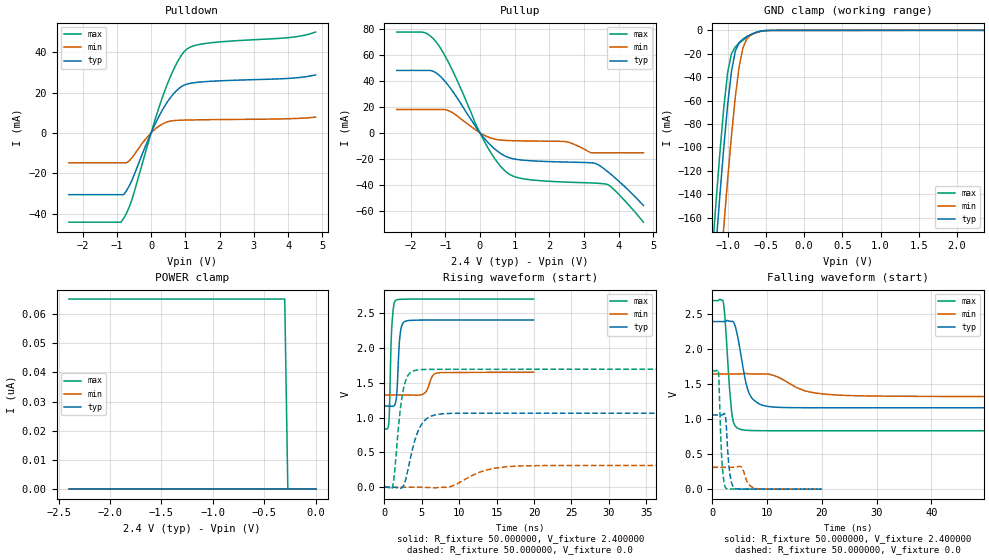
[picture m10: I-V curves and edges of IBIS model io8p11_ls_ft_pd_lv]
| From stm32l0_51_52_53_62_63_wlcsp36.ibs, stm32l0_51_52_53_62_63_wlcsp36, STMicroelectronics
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|   Model io8p11_ls_ft_pd_lv
[Model]  io8p11_ls_ft_pd_lv
Model_type I/O
Polarity   Non-Inverting
Enable   Active-Low
Vinl =   0.720000V
Vinh =   1.680000V
Vmeas =  1.200000V
Cref =   50.000000pF
Rref =   100.000000M
Vref =   0.0V
C_comp   4.521100pF   4.438000pF   4.578000pF
[Temperature Range]   25.000000   0.105000k   -40.000000
[Pullup Reference]   2.400000V   1.650000V   2.700000V
[Pulldown Reference]   0.0V   0.0V   0.0V
[POWER Clamp Reference]   2.400000V   1.650000V   2.700000V
[GND Clamp Reference]   0.0V   0.0V   0.0V
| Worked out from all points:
|   slope of the pulldown table from 0 to 0.36 V, typ, clamps not added: 29.5 ohm
|   slope of the pullup table from 0 to 0.36 V, typ, clamps not added: 33.2 ohm
|   GND clamp passes 1 mA (typ) near -0.59 V on its own axis
|   rising waveform, R_fixture 50.000000, V_fixture 2.400000: 20-80 % time 365ps typ, 690ps min, 304ps max; typ from 1.17 V to 2.4 V
|   rising waveform, R_fixture 50.000000, V_fixture 0.0: 20-80 % time 1.62ns typ, 3.85ns min, 984ps max; typ from 0 V to 1.06 V
|   falling waveform, R_fixture 50.000000, V_fixture 2.400000: 20-80 % time 1.82ns typ, 5.41ns min, 983ps max; typ from 2.4 V to 1.17 V
|   falling waveform, R_fixture 50.000000, V_fixture 0.0: 20-80 % time 621ps typ, 1.01ns min, 515ps max; typ from 1.06 V to 0 V
[Pulldown]
|Voltage   I(typ)   I(min)   I(max)
-2.4V     -30.64mA   -14.84mA   -44.29mA
-880mV    -30.64mA   -14.84mA   -44.29mA
-800mV    -30.64mA   -14.84mA   -42.37mA
-560mV    -23.52mA   -12.34mA   -33.09mA
0V        -765.1nA   -61.09nA   -2.527uA
400mV     13.38mA    4.998mA    20.91mA
720mV     20.62mA    6.178mA    33.69mA
880mV     22.92mA    6.306mA    38.42mA
1.04V     24.19mA    6.384mA    41.49mA
1.6V      25.46mA    6.543mA    44.41mA
4.08V     27.12mA    7.07mA     47.39mA
4.8V      28.77mA    7.815mA    50.01mA
[Pullup]
|Voltage   I(typ)   I(min)   I(max)
-2.4V     48.08mA    17.97mA    77.6mA
-1.6V     48.08mA    17.97mA    77.22mA
-1.28V    46.45mA    17.97mA    70.55mA
-880mV    35.37mA    16.81mA    52.8mA
160mV     -5.286mA   -2.324mA   -8.223mA
480mV     -13.62mA   -5.102mA   -21.86mA
800mV     -18.73mA   -5.909mA   -31mA
1.28V     -21.13mA   -6.237mA   -35.54mA
2.48V     -22.51mA   -6.819mA   -37.93mA
3.36V     -23.83mA   -15.36mA   -38.77mA
3.76V     -31.49mA   -15.36mA   -41.07mA
4.72V     -56mA      -15.36mA   -68.83mA
[GND_clamp]
|Voltage   I(typ)   I(min)   I(max)
-2.4V     -1.379A    -1.445A    -1.349A
-1.2V     -225.9mA   -297.5mA   -189.2mA
-1.15V    -182mA     -253.1mA   -145.3mA
-1.1V     -139.6mA   -209.7mA   -103.5mA
-1.05V    -99.62mA   -167.6mA   -65.7mA
-1V       -63.68mA   -127.3mA   -35.9mA
-950mV    -35mA      -89.93mA   -19.88mA
-900mV    -17.68mA   -57.02mA   -14.13mA
-850mV    -10.5mA    -31.19mA   -11.01mA
-750mV    -5.3mA     -7.337mA   -6.005mA
-450mV    -43.41uA   -101.2uA   -21.28uA
2.35V     52.68uA    50.02uA    36.83uA
[POWER_clamp]
|Voltage   I(typ)   I(min)   I(max)
-2.4V     0A         0A         65.17nA
-300mV    0A         0A         65.17nA
-270mV    0A         0A         0A
0V        0A         0A         0A
[Ramp]
| variable   typ   min   max
dV/dt_r  0.63713/1.61823n   0.18752/3.84950n   1.01518/0.97852n
dV/dt_f  0.74040/1.81884n   0.19362/5.38899n   1.11767/0.98038n
R_load = 50.000000
[Rising Waveform]
R_fixture= 50.000000
V_fixture= 2.400000
V_fixture_min= 1.650000
V_fixture_max= 2.700000
|time   V(typ)   V(min)   V(max)
0s        1.165V     1.324V     835.9mV
600.6ps   1.164V     1.324V     938.4mV
961ps     1.16V      1.324V     2.255V
1.481ns   1.209V     1.324V     2.679V
1.682ns   1.389V     1.324V     2.689V
2.082ns   2.177V     1.324V     2.695V
2.683ns   2.375V     1.324V     2.697V
5.205ns   2.398V     1.338V     2.699V
7.047ns   2.399V     1.638V     2.699V
19.94ns   2.399V     1.649V     2.699V
[Rising Waveform]
R_fixture= 50.000000
V_fixture= 0.0
V_fixture_min= 0.0
V_fixture_max= 0.0
|time   V(typ)   V(min)   V(max)
0s        63.36uV    12.74uV    531.9uV
1.126ns   -151.4uV   9.604uV    28.27mV
2.002ns   -20.43mV   22.63uV    1.001V
2.503ns   11.79mV    99.44uV    1.389V
3.128ns   243.6mV    98.4uV     1.601V
4.129ns   693.8mV    62.69uV    1.676V
5.506ns   971mV      -2.231mV   1.69V
7.758ns   1.054V     -1.515mV   1.692V
16.52ns   1.062V     296.3mV    1.692V
62.31ns   1.062V     312.5mV    1.692V
[Falling Waveform]
R_fixture= 50.000000
V_fixture= 2.400000
V_fixture_min= 1.650000
V_fixture_max= 2.700000
|time   V(typ)   V(min)   V(max)
0s        2.399V     1.649V     2.699V
2.002ns   2.398V     1.648V     2.673V
2.252ns   2.399V     1.648V     2.498V
3.504ns   2.401V     1.648V     1.121V
4.004ns   2.369V     1.648V     927.9mV
4.88ns    2.073V     1.648V     863.5mV
6.632ns   1.387V     1.651V     840.8mV
9.635ns   1.192V     1.648V     836.4mV
21.02ns   1.165V     1.356V     835.9mV
62.31ns   1.165V     1.324V     835.9mV
[Falling Waveform]
R_fixture= 50.000000
V_fixture= 0.0
V_fixture_min= 0.0
V_fixture_max= 0.0
|time   V(typ)   V(min)   V(max)
0s        1.062V     312.5mV    1.692V
1.121ns   1.062V     312.5mV    1.669V
1.522ns   1.061V     312.5mV    772.9mV
1.762ns   1.063V     312.5mV    385.5mV
2.482ns   973.1mV    312.5mV    13.17mV
3.163ns   237.9mV    312.2mV    2.666mV
4.044ns   18.6mV     314.7mV    1.752mV
5.285ns   1.812mV    318.3mV    1.024mV
7.928ns   541uV      8.99mV     645.8uV
19.94ns   63.36uV    12.74uV    531.9uV
